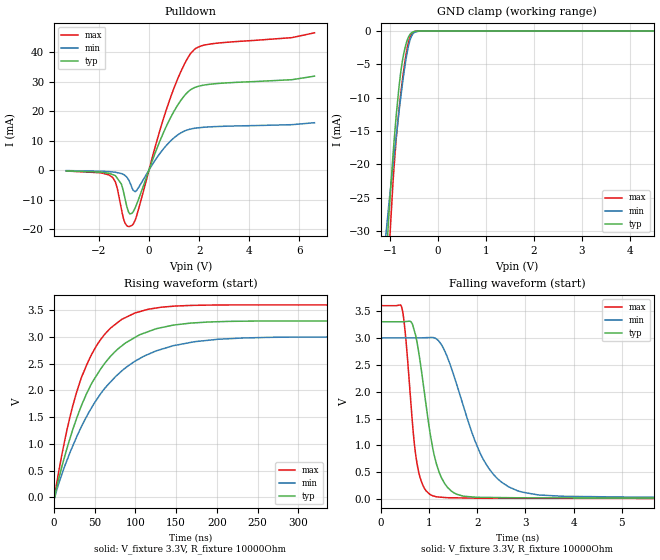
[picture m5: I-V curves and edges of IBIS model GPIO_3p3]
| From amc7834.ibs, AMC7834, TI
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|   Model
[Model]   GPIO_3p3
Model_type   I/O_open_drain
Polarity   Non-Inverting
Enable   Active-Low
Vinl = 0.9
Vinh = 2.31
Vmeas = 1.65
Vref = 3.3
Cref = 1pF
Rref = 10000
|   typ   min   max
C_comp   2.622pF   2.415pF   2.744pF
[Voltage Range]   3.3   3   3.6
[Temperature Range]   27   125   -40
[Pullup Reference]   3.3   3   3.6
[Pulldown Reference]   0   0   0
[Power Clamp Reference]   3.3   3   3.6
[GND Clamp Reference]   0   0   0
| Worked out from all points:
|   slope of the pulldown table from 0 to 0.495 V, typ, clamps not added: 44.7 ohm
|   GND clamp passes 1 mA (typ) near -0.63 V on its own axis
|   falling waveform, V_fixture 3.3V, R_fixture 10000Ohm: 20-80 % time 348ps typ, 733ps min, 210ps max; typ from 3.3 V to 0.013 V
|   rising waveform, V_fixture 3.3V, R_fixture 10000Ohm: 20-80 % time 58.2ns typ, 72.3ns min, 45.3ns max; typ from 0.013 V to 3.3 V
[Pulldown]
|   Voltage   I(typ)   I(min)   I(max)
-3.3V     -288uA     -180.1uA   -326.1uA
-1.459V   -1.511mA   -638.7uA   -2.466mA
-1.27V    -2.709mA   -867.2uA   -5.978mA
-1.102V   -4.724mA   -1.179mA   -13.11mA
-948.3mV  -9.933mA   -1.917mA   -18.09mA
-815.1mV  -14.24mA   -3.245mA   -19.2mA
-676.5mV  -14.66mA   -6.017mA   -18.78mA
-498.3mV  -11.76mA   -6.981mA   -15.68mA
709.5mV   15.19mA    8.525mA    20.95mA
1.68V     27.4mA     13.98mA    39.8mA
2.373V    29.09mA    14.65mA    42.72mA
6.6V      31.9mA     16.08mA    46.62mA
[GND Clamp]
|   Voltage   I(typ)   I(min)   I(max)
-3.3V     -354.2mA   -256.1mA   -449.5mA
-1.092V   -34.88mA   -30.58mA   -43.59mA
-1.023V   -26.92mA   -25.49mA   -32.83mA
-1.013V   -25.84mA   -24.8mA    -31.44mA
-943.8mV  -18.66mA   -20.13mA   -22.76mA
-874.5mV  -12.53mA   -15.71mA   -16.03mA
-785.4mV  -6.387mA   -10.18mA   -9.678mA
-716.1mV  -3.306mA   -6.343mA   -5.67mA
-646.8mV  -1.391mA   -3.21mA    -2.543mA
-587.4mV  -498.9uA   -1.363mA   -898.9uA
-528mV    -135.4uA   -438.5uA   -211.3uA
6.6V      0A         0A         0A
[POWER Clamp]
|   Voltage   I(typ)   I(min)   I(max)
-3.3V     0A         0A         0A
0V        0A         0A         0A
6.6V      0A         0A         0A
[Ramp]
R_load = 10000
|   typ   min   max
dV/dt_r   1.97197/5.82335e-08   1.78764/7.22784e-08   2.15351/4.52764e-08
dV/dt_f   1.97197/3.4806e-10   1.78766/7.33258e-10   2.15351/2.105e-10
[Falling Waveform]
V_fixture = 3.3V
V_fixture_min = 3V
V_fixture_max = 3.6V
R_fixture = 10000Ohm
C_fixture = 0F
|   Time   V(typ)   V(min)   V(max)
0s        3.3V       3V         3.6V
440.4ps   3.3V       3V         3.556V
712.4ps   3.086V     3V         918.8mV
879.2ps   2.163V     3.002V     249.3mV
1.08ns    941.8mV    3.007V     64.38mV
1.258ns   403.3mV    2.878V     38.1mV
2.055ns   36.06mV    873.1mV    19.53mV
3.297ns   26.38mV    78.78mV    17.96mV
12.04ns   15.35mV    26.61mV    10.84mV
500ns     13.39mV    20.75mV    10.8mV
[Rising Waveform]
V_fixture = 3.3V
V_fixture_min = 3V
V_fixture_max = 3.6V
R_fixture = 10000Ohm
C_fixture = 0F
|   Time   V(typ)   V(min)   V(max)
0s        13.39mV    20.75mV    10.8mV
533.7ps   1.075mV    20.99mV    -23.95mV
19.6ns    1.092V     830.2mV    1.492V
27.48ns   1.457V     1.113V     1.943V
40.2ns    1.941V     1.512V     2.473V
62.66ns   2.512V     2.043V     3.056V
99.66ns   2.993V     2.548V     3.45V
146.4ns   3.222V     2.837V     3.576V
201.1ns   3.286V     2.957V     3.598V
500ns     3.3V       3V         3.6V
